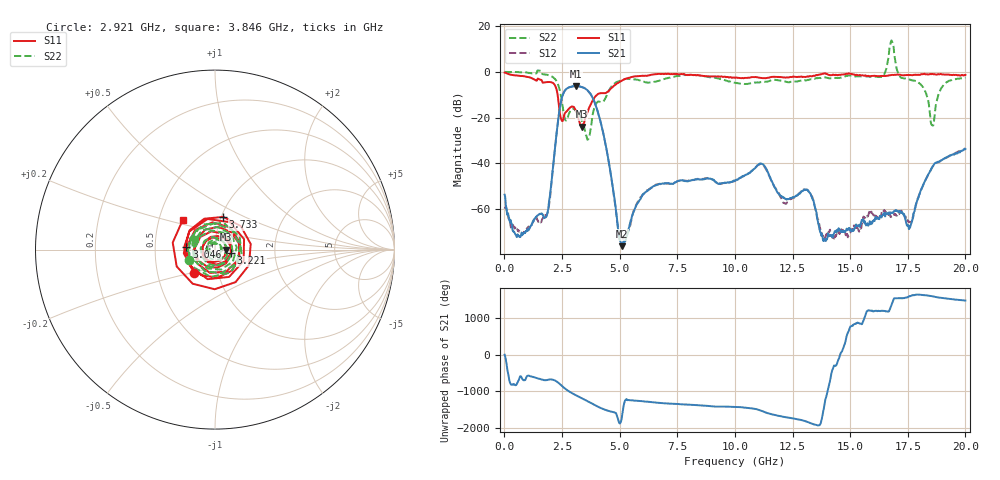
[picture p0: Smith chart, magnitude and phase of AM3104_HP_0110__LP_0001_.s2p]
!Created with skrf (http://scikit-rf.org).
# Hz S RI R 50.0
!freq ReS11 ImS11 ReS21 ImS21 ReS12 ImS12 ReS22 ImS22
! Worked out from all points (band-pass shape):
!   1601 points, 10 MHz to 20 GHz, reference 50 ohm
!   highest |S21| = -6.20 dB at 3.108 GHz (marker M1); lowest = -76.1 dB at 5.095 GHz (marker M2)
!   |S21| within 3 dB of the highest: 2.57 GHz to 3.709 GHz (1.139 GHz wide, 36.3 % of centre)
!   lowest |S11| = -24.0 dB at 3.346 GHz (marker M3), VSWR 1.13, Z = 56.7 - j0.139 ohm
!   |S11| at or under -10 dB: 2.309 GHz to 4.026 GHz (1.718 GHz wide, 54.2 % of centre)
!   |S22| runs from -29.6 to 13.7 dB; largest |S21 - S12| = 0.027
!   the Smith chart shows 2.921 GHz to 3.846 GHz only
!   S11 on the Smith chart (normalised r, x): 2.921 GHz: 0.77, -0.21; 3.046 GHz: 0.72, +0.02; 3.221 GHz: 1.19, -0.05; 3.733 GHz: 1.02, +0.39; 3.846 GHz: 0.66, +0.23
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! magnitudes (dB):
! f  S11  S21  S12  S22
! 10 MHz  -0.3  -53.6  -59.8  0.0
! 597.2 MHz  -1.7  -71.2  -69.0  -0.1
! 1.797 GHz  -4.5  -63.5  -63.0  -1.2
! 2.446 GHz  -20.1  -13.5  -13.5  -10.1
! 2.921 GHz  -15.1  -6.4  -6.5  -16.3
! 3.046 GHz  -15.9  -6.3  -6.3  -16.4
! 3.108 GHz  -17.0  -6.2  -6.2  -17.3
! 3.221 GHz  -20.8  -6.3  -6.4  -18.7
! 3.346 GHz  -24.0  -6.6  -6.6  -20.7
! 3.733 GHz  -14.5  -9.5  -9.6  -25.4
! 3.846 GHz  -12.2  -11.7  -11.7  -17.9
! 5.095 GHz  -3.8  -76.1  -72.5  -3.7
! 6.682 GHz  -0.9  -49.1  -49.0  -4.0
! 10.01 GHz  -2.6  -47.5  -47.7  -4.8
! 11.15 GHz  -2.8  -40.1  -40.3  -4.5
! 12.14 GHz  -2.5  -55.1  -57.2  -4.1
! 13.34 GHz  -2.0  -54.7  -54.3  -3.3
! 13.9 GHz  -0.7  -73.1  -72.4  -2.4
! 16.68 GHz  -1.5  -61.7  -62.5  7.2
! 17.59 GHz  -1.5  -67.4  -65.4  -3.5
! 18.56 GHz  -0.9  -41.5  -41.5  -23.3
! 20 GHz  -1.4  -33.7  -33.5  -2.5
